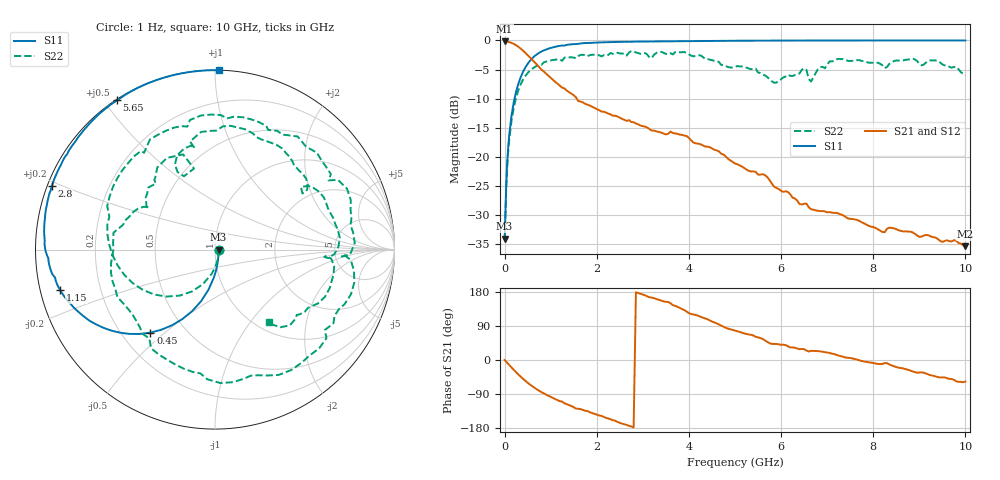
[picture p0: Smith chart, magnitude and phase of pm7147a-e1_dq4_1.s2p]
# GHz S DB R 50
! S-Parameters data
! Freq  dbS11  angS11  dbS21  angS21  dbS12  angS12  dbS22  angS22
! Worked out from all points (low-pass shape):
!   279 points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, 1 Hz to 10 GHz, reference 50 ohm
!   highest |S21| = -0.17 dB at 316.2 Hz (marker M1); lowest = -35.3 dB at 10 GHz (marker M2)
!   |S21| within 3 dB of the highest: start of sweep to 580.6 MHz
!   lowest |S11| = -34.1 dB at 251.2 Hz (marker M3), VSWR 1.04, Z = 52 - j2.99e-05 ohm
!   |S11| at or under -10 dB: start of sweep to 215.3 MHz
!   |S22| runs from -34.1 to -1.8 dB; largest |S21 - S12| = 0
!   S11 on the Smith chart (normalised r, x): 1 Hz: 1.04, -0.00; 450 MHz: 0.32, -0.45; 1.15 GHz: 0.06, -0.13; 2.8 GHz: 0.01, +0.19; 5.65 GHz: 0.00, +0.54; 10 GHz: 0.00, +1.03
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1e-09  -34.05 -0.0  -0.17 -0.0  -0.17 -0.0  -34.05 -0.0
2.512e-07  -34.05 -0.0  -0.17 -0.0  -0.17 -0.0  -34.05 -0.0
3.162e-07  -34.05 -0.0  -0.17 -0.0  -0.17 -0.0  -34.05 -0.0
0.06309573  -20.10 -84.2  -0.22 -8.4  -0.22 -8.4  -20.94 -87.5
0.15  -12.88 -99.2  -0.42 -19.8  -0.42 -19.8  -13.79 -109.4
0.45  -4.64 -127.9  -2.13 -55.1  -2.13 -55.1  -6.10 -158.0
0.85  -1.72 -153.1  -5.32 -87.9  -5.32 -87.9  -3.77 158.0
1.15  -1.00 -165.3  -7.44 -106.0  -7.44 -106.0  -3.24 131.1
1.7  -0.47 179.4  -10.65 -131.7  -10.65 -131.7  -2.47 91.6
2.3  -0.28 167.0  -12.70 -156.8  -12.70 -156.8  -2.15 53.8
2.8  -0.21 158.6  -14.04 -178.1  -14.04 -178.1  -1.88 20.0
3.35  -0.17 150.5  -15.72 158.8  -15.72 158.8  -1.97 -13.3
3.9  -0.14 143.2  -16.34 131.7  -16.34 131.7  -2.00 -57.5
4.25  -0.11 138.9  -17.83 114.3  -17.83 114.3  -2.57 -87.7
5.05  -0.05 129.6  -21.25 76.1  -21.25 76.1  -4.38 -154.1
5.65  -0.04 123.2  -23.13 51.7  -23.13 51.7  -6.00 155.2
6.55  -0.01 114.5  -28.03 25.1  -28.03 25.1  -5.05 108.5
6.7  -0.01 113.1  -29.06 24.1  -29.06 24.1  -6.37 115.8
7.25  -0.01 108.3  -29.73 11.5  -29.73 11.5  -3.16 82.7
8.35  -0.00 99.6  -32.16 -11.9  -32.16 -11.9  -4.01 34.4
9.25  -0.00 93.3  -33.66 -40.3  -33.66 -40.3  -3.41 -11.7
10  -0.00 88.6  -35.33 -56.9  -35.33 -56.9  -5.98 -53.4
